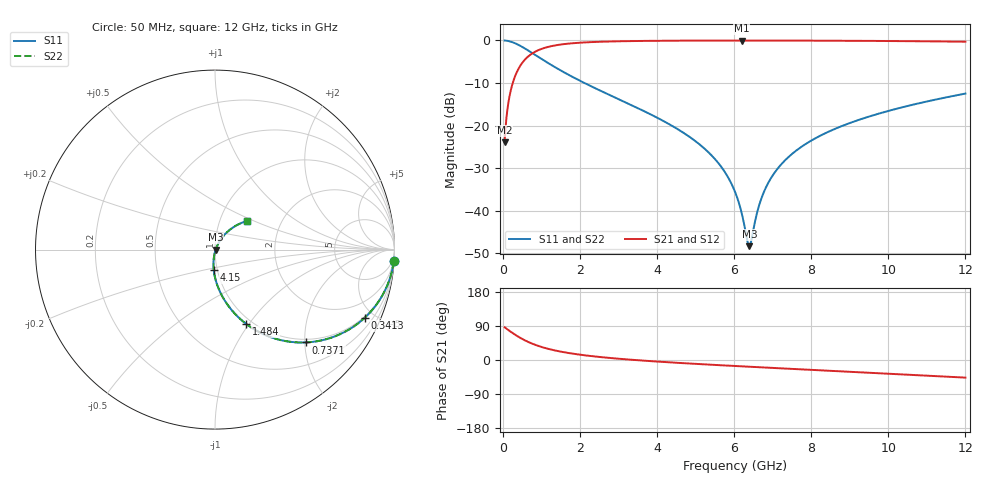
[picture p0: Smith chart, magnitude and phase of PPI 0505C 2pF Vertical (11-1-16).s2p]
# GHz S MA R 50
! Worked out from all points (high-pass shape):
!   1601 points, 50 MHz to 12 GHz, reference 50 ohm
!   highest |S21| = -0.04 dB at 6.197 GHz (marker M1); lowest = -23.9 dB at 50 MHz (marker M2)
!   |S21| within 3 dB of the highest: 771.5 MHz to end of sweep
!   lowest |S11| = -48.3 dB at 6.398 GHz (marker M3), VSWR 1.01, Z = 50.4 - j0.105 ohm
!   |S11| at or under -10 dB: 2.119 GHz to end of sweep
!   |S22| runs from -48.3 to 0.0 dB; largest |S21 - S12| = 0
!   S11 on the Smith chart (normalised r, x): 50 MHz: 1, -30; 341.3 MHz: 0.93, -4.42; 737.1 MHz: 0.93, -2.03; 1.484 GHz: 0.93, -0.97; 4.15 GHz: 0.96, -0.22; 12 GHz: 1.34, +0.45
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0.05  0.998 -3.8  0.0636 86.2  0.0636 86.2  0.998 -3.8
0.1844375  0.9733 -13.8  0.229 76.2  0.229 76.2  0.9733 -13.8
0.3412812  0.9164 -24.5  0.3996 65.4  0.3996 65.4  0.9164 -24.5
0.737125  0.7241 -45.6  0.6883 44.3  0.6883 44.3  0.7241 -45.6
1.080688  0.5769 -57.6  0.815 32.2  0.815 32.2  0.5769 -57.6
1.484  0.449 -67.2  0.8914 22.5  0.8914 22.5  0.449 -67.2
2.044156  0.3288 -76.1  0.9419 13.5  0.9419 13.5  0.3288 -76.1
4.038312  0.1215 -92.9  0.9892 -4.3  0.9892 -4.3  0.1215 -92.9
4.150344  0.1142 -93.5  0.9901 -5.0  0.9901 -5.0  0.1142 -93.5
5.360281  0.04739 -98.0  0.995 -12.2  0.995 -12.2  0.04739 -98.0
5.748656  0.02905 -97.2  0.9956 -14.4  0.9956 -14.4  0.02905 -97.2
6.025  0.01668 -93.0  0.9958 -15.8  0.9958 -15.8  0.01668 -93.0
6.196781  0.009435 -83.2  0.9958 -16.7  0.9958 -16.7  0.009435 -83.2
6.338687  0.004536 -50.2  0.9958 -17.5  0.9958 -17.5  0.004536 -50.2
6.398438  0.003835 -15.8  0.9958 -17.8  0.9958 -17.8  0.003835 -15.8
6.450719  0.004527 13.7  0.9957 -18.1  0.9957 -18.1  0.004527 13.7
6.68225  0.01286 53.0  0.9956 -19.3  0.9956 -19.3  0.01286 53.0
6.951125  0.02385 59.7  0.9953 -20.6  0.9953 -20.6  0.02385 59.7
7.391781  0.04187 61.4  0.9945 -22.9  0.9945 -22.9  0.04187 61.4
8.019156  0.06726 60.2  0.9929 -26.0  0.9929 -26.0  0.06726 60.2
10.01331  0.149 52.0  0.9831 -36.1  0.9831 -36.1  0.149 52.0
12  0.2374 42.1  0.9647 -46.5  0.9647 -46.5  0.2374 42.1
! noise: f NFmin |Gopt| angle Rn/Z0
0.05  0.0008917  0.9504  1.592  0.004037
1.372  0.005523  0.7549  5.112  0.004544
2.701  0.008613  0.6995  8.478  0.005579
4.031  0.01134  0.6664  11.86  0.006453
5.36  0.01391  0.6442  15.21  0.007278
6.682  0.01643  0.6293  18.49  0.008108
8.012  0.01898  0.6196  21.71  0.008993
9.341  0.02163  0.6142  24.88  0.009962
10.67  0.02441  0.6127  27.98  0.01106
12  0.02739  0.6145  31.02  0.01232
